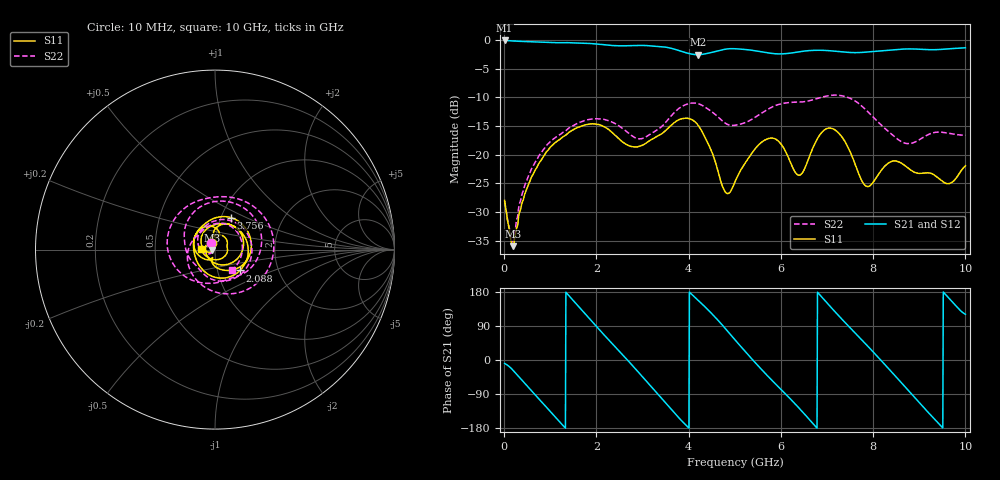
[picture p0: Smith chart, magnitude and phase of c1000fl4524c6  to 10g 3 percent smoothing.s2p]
!Agilent Technologies,N5234A,MY52241123,A.10.00.00
!Agilent N5234A: A.10.00.00
!Date: Wednesday, April 17, 2019 13:52:14
!Correction: S11(Full 2 Port(1,2))
!S21(Full 2 Port(1,2))
!S12(Full 2 Port(1,2))
!S22(Full 2 Port(1,2))
!S2P File: Measurements: S11, S21, S12, S22:
# Hz S  dB  R 50
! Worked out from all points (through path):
!   1001 points, 10 MHz to 10 GHz, reference 50 ohm
!   highest |S21| = -0.08 dB at 10 MHz (marker M1); lowest = -2.5 dB at 4.196 GHz (marker M2)
!   group delay of S21, straight-line fit = 366 ps
!   lowest |S11| = -35.9 dB at 189.8 MHz (marker M3), VSWR 1.03, Z = 48.5 - j0.328 ohm
!   |S11| at or under -10 dB: start of sweep to end of sweep
!   |S22| runs from -35.2 to -9.6 dB; largest |S21 - S12| = 0.0016
!   S11 on the Smith chart (normalised r, x): 10 MHz: 0.96, +0.07; 2.088 GHz: 1.28, -0.31; 3.756 GHz: 1.11, +0.41; 10 GHz: 0.85, +0.01
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1e7  -27.97 117.3  -0.08 -9.2  -0.06 -9.1  -28.05 120.4
1.8982e8  -35.93 -167.8  -0.17 -26.8  -0.16 -26.8  -35.15 -157.4
7.9921e8  -21.01 150.5  -0.37 -109.0  -0.37 -108.9  -19.72 157.0
1.25875e9  -16.96 86.7  -0.47 -170.6  -0.47 -170.6  -16.18 96.3
1.67833e9  -15.00 27.9  -0.53 132.4  -0.53 132.5  -14.24 41.7
2.08792e9  -14.81 -39.8  -0.76 76.8  -0.75 76.8  -13.74 -17.4
2.71729e9  -18.48 -148.7  -0.99 -6.0  -0.98 -6.0  -16.38 -112.5
3.34666e9  -16.66 122.5  -1.14 -92.0  -1.14 -92.1  -15.51 173.1
3.75625e9  -14.02 63.6  -1.75 -148.5  -1.75 -148.5  -12.14 113.3
4.19581e9  -14.75 -23.1  -2.55 158.6  -2.55 158.6  -11.07 33.3
4.67533e9  -24.02 -106.8  -1.82 99.7  -1.82 99.7  -13.69 -40.0
5.005e9  -24.71 -112.2  -1.52 53.2  -1.52 53.2  -14.85 -74.2
5.42458e9  -19.13 -177.8  -1.85 -4.5  -1.85 -4.5  -13.55 -123.8
5.94406e9  -17.62 99.3  -2.42 -70.6  -2.42 -70.5  -11.25 164.1
6.67333e9  -19.18 91.4  -1.81 -164.7  -1.81 -164.8  -10.46 79.1
7.003e9  -15.41 45.7  -1.83 150.1  -1.83 150.1  -9.75 41.7
7.47253e9  -18.98 -44.6  -2.16 88.5  -2.16 88.5  -10.07 -22.8
7.97203e9  -25.09 156.5  -2.01 25.1  -2.01 25.1  -13.19 -103.3
8.34166e9  -21.39 76.0  -1.75 -23.7  -1.75 -23.7  -16.02 -167.1
8.96104e9  -23.21 14.1  -1.58 -107.5  -1.58 -107.5  -17.57 109.5
9.48052e9  -24.50 -64.2  -1.63 -175.4  -1.63 -175.4  -16.07 34.4
1e10  -21.93 176.8  -1.35 120.7  -1.36 120.6  -16.60 -49.8
